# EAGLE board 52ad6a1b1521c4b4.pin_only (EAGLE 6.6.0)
REV: C

Size 26.67 x 20.32 mm. Coordinates in mm from the lower left corner, seen from the top.
Outline: 2.54,20.32 24.13,20.32 arc-90 26.67,17.78 26.67,2.54 arc-90 24.13,0 2.54,0 arc-90 0,2.54 0,17.78 arc-90 2.54,20.32
Copper layers (1*16): Top 0.035mm / dielectric 1.5mm / Bottom 0.035mm
Design rules "adafruit *": minimum track width 8mil, minimum drill 15.5mil, track to track 8mil, track to pad 8mil, pad to pad 8mil, via to via 8mil, smd to smd 8mil, copper to edge 10mil, drill to drill 8mil, minimum pad ring 10mil, minimum via ring 8mil, stop-mask expansion 2mil, vias tented up to drill 20mil, thermal gap 10mil

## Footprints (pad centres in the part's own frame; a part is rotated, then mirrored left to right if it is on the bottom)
0805-NO = smd 1.3 x 1.5: 1 -0.95,0; 2 0.95,0
0805_10MGAP = smd 1.2 x 1.5: 1 -1.05,0; 2 1.05,0
SOD-323 = smd 1.35 x 0.8: A 1.27,0; C -1.27,0
FIDUCIAL_1MM = smd 1 x 1: 1 0,0
1X06_ROUND_76 = drill 1 pad 1.93: 1 -6.35,0; 2 -3.81,0; 3 -1.27,0; 4 1.27,0; 5 3.81,0; 6 6.35,0
1X04_ROUND_76 = drill 1 pad 1.93: 1 -3.81,0; 2 -1.27,0; 3 1.27,0; 4 3.81,0
SOT23-WIDE = smd 1 x 1.2: 1 -0.95,-1; 2 0.95,-1; 3 0,1
_0805MP = smd 1.2 x 1.3: 1 -1.016,0; 2 1.016,0
SOT23-5 = smd 0.55 x 1.2: 1 -0.95,-1.3; 2 0,-1.3; 3 0.95,-1.3; 4 0.95,1.3; 5 -0.95,1.3
BNO055 = smd 0.25 x 0.475: 1 -2.25,1.562; 6 -2.25,-1.562; 7 -1.75,-1.562; 8 -1.25,-1.562; 9 -0.75,-1.562; 10 -0.25,-1.562; 11 0.25,-1.562; 12 0.75,-1.562; 13 1.25,-1.562; 14 1.75,-1.562; 15 2.25,-1.562; 20 2.25,1.562; 21 1.75,1.562; 22 1.25,1.562; 23 0.75,1.562; 24 0.25,1.562; 25 -0.25,1.562; 26 -0.75,1.562; 27 -1.25,1.562; 28 -1.75,1.562 | smd 0.375 x 0.25: 2 -2.312,0.75; 3 -2.312,0.25; 4 -2.312,-0.25; 5 -2.312,-0.75; 16 2.312,-0.75; 17 2.312,-0.25; 18 2.312,0.25; 19 2.312,0.75
MOUNTINGHOLE_2.5_PLATED_THICK = drill 2.5 pad 4: P$1 0,0
CRYSTAL_8X3.8 = smd 1.3 x 1.9: P$1 -2.75,-1.6; P$2 2.75,-1.6; P$3 2.75,1.6; P$4 -2.75,1.6

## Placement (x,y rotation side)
C1  22pF  [0805-NO]  7.62,8.13 0 top
C2  22pF  [0805-NO]  7.11,15.62 0 top
C3  0.1uF  [0805-NO]  17.53,8.76 180 top
C4  0.1uF  [0805_10MGAP]  12.45,5.21 90 top
C5  10uF  [0805-NO]  4.32,7.11 90 top
C6  10uF  [0805_10MGAP]  10.54,5.33 270 top
D1  1n4148  [SOD-323]  17.65,10.79 180 top
FID1  FIDUCIAL""  [FIDUCIAL_1MM]  20.83,18.92 0 top
FID2  FIDUCIAL""  [FIDUCIAL_1MM]  1.65,5.84 0 top
JP1  [1X06_ROUND_76]  13.34,1.27 0 top
JP2  [1X04_ROUND_76]  13.34,19.05 0 top
Q1  BSS138  [SOT23-WIDE]  20.95,13.72 0 top
Q2  BSS138  [SOT23-WIDE]  20.7,5.21 180 top
R3  10K  [0805-NO]  11.43,15.37 270 top
R4  10K  [0805-NO]  13.34,15.24 270 top
R5  10K  [0805-NO]  17.27,15.88 0 top
R6  10K  [0805-NO]  21.46,10.92 180 top
R7  10K  [0805-NO]  21.21,7.87 0 top
R8  10K  [_0805MP]  14.61,5.33 90 top
R9  10K  [_0805MP]  17.91,5.33 90 top
R10  10K  [0805-NO]  17.4,13.21 0 top
U1  MIC5225-3.3  [SOT23-5]  7.49,5.33 270 top
U$2  BNO055  [BNO055]  13.34,10.16 90 top
U$3  [PCBFEAT-REV-040]  24.64,10.92 0 bottom
U$28  [ADAFRUIT_TEXT_20MM]  26.42,3.05 0 bottom
U$29  MOUNTINGHOLE2.5_THICK  [MOUNTINGHOLE_2.5_PLATED_THICK]  2.54,17.78 0 top
U$30  MOUNTINGHOLE2.5_THICK  [MOUNTINGHOLE_2.5_PLATED_THICK]  2.54,2.54 0 top
U$31  MOUNTINGHOLE2.5_THICK  [MOUNTINGHOLE_2.5_PLATED_THICK]  24.13,17.78 0 top
U$32  MOUNTINGHOLE2.5_THICK  [MOUNTINGHOLE_2.5_PLATED_THICK]  24.13,2.54 0 top
U$33  [ADAFRUIT_2.5MM]  5.33,17.27 0 top
Y1  32.768kHz  [CRYSTAL_8X3.8]  6.1,11.81 180 top

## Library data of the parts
C1-C6 D1 JP1 JP2 Q1 Q2 R3-R10 U1 U$2 U$3 U$28 U$33 Y1 = microbuilder
FID1 FID2 U$29-U$32 = microbuilder; BOM: EXCLUDE

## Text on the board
tPlace: PS0 | PS1 | INT | ADR | BNO055 | 9-Axis Abs. / Orientation | Vin | 3vo | GND | SDA | SCL | RST
bPlace: BNO055 | Vin:3-5V DC, 3V logic / SDA/SCL/RST: 5V ok | 3-Axis Accel+Gyro+Mag / w/Quaternion, Euler / Heading, etc. I2C Out

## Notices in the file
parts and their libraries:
microbuilder: This work is placed in the public domain, and may be freely used for commercial and non-commercial work with the following conditions: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
